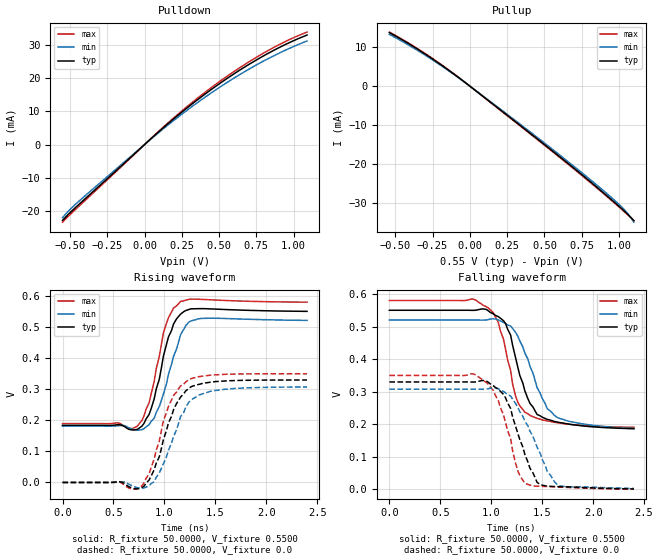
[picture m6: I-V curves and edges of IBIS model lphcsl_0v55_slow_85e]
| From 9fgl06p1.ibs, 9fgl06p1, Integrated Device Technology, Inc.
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[Model]   lphcsl_0v55_slow_85e
Model_type Output
Polarity   Inverting
Enable   Active-High
Vmeas =  0.4000V
Cref =   2.0000pF
Rref =   0.0
Vref =   0.4000V
C_comp   1.1000pF   1.0000pF   1.2000pF
[Temperature Range]   25.0000   85.0000   -40.0
[Voltage Range]   0.5500V   0.5200V   0.5800V
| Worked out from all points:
|   slope of the pulldown table from 0 to 0.083 V, typ, clamps not added: 24.5 ohm
|   slope of the pullup table from 0 to 0.083 V, typ, clamps not added: 33.4 ohm
|   rising waveform, R_fixture 50.0000, V_fixture 0.5500: 20-80 % time 164ps typ, 185ps min, 153ps max; typ from 0.184 V to 0.551 V
|   rising waveform, R_fixture 50.0000, V_fixture 0.0: 20-80 % time 212ps typ, 224ps min, 196ps max; typ from 0 V to 0.33 V
|   falling waveform, R_fixture 50.0000, V_fixture 0.5500: 20-80 % time 209ps typ, 258ps min, 182ps max; typ from 0.55 V to 0.186 V
|   falling waveform, R_fixture 50.0000, V_fixture 0.0: 20-80 % time 215ps typ, 272ps min, 192ps max; typ from 0.33 V to 0.002 V
[Pulldown]
|Voltage   I(typ)   I(min)   I(max)
-550mV    -22.86mA   -22.05mA   -23.4mA
-490mV    -20.12mA   -19.14mA   -20.7mA
-430mV    -17.63mA   -16.68mA   -18.17mA
50mV      2.058mA    1.922mA    2.135mA
230mV     9.045mA    8.465mA    9.373mA
410mV     15.37mA    14.42mA    15.91mA
590mV     21.04mA    19.77mA    21.74mA
770mV     26.03mA    24.5mA     26.86mA
930mV     29.87mA    28.16mA    30.76mA
1.09V     33.04mA    31.25mA    33.93mA
[Pullup]
|Voltage   I(typ)   I(min)   I(max)
-540mV    13.79mA    13.35mA    13.94mA
-360mV    9.757mA    9.424mA    9.891mA
-180mV    5.143mA    4.956mA    5.227mA
-20mV     596.4uA    573.5uA    607.4uA
340mV     -10.2mA    -9.898mA   -10.34mA
640mV     -19.35mA   -18.88mA   -19.54mA
920mV     -28.28mA   -27.72mA   -28.48mA
1.04V     -32.36mA   -32.02mA   -32.52mA
1.1V      -34.69mA   -35.06mA   -34.66mA
[Ramp]
| variable   typ   min   max
dV/dt_r  0.1981/0.2090n   0.1846/0.2327n   0.2101/0.1963n
dV/dt_f  0.2182/0.2310n   0.1998/0.2513n   0.2335/0.2061n
R_load = 50.0000
[Rising Waveform]
R_fixture= 50.0000
V_fixture= 0.5500
V_fixture_min= 0.5200
V_fixture_max= 0.5800
|time   V(typ)   V(min)   V(max)
0s        184mV      181.7mV    189.6mV
730ps     170.5mV    168.3mV    180.5mV
850ps     219.2mV    186.3mV    256.9mV
900ps     269.4mV    207.1mV    325.8mV
1.02ns    444.5mV    316.9mV    512.3mV
1.09ns    510.7mV    406.8mV    562.1mV
1.16ns    542.8mV    477.1mV    583.6mV
1.24ns    557.4mV    517mV      589.9mV
1.36ns    560.2mV    528.6mV    590.2mV
2.4ns     551.4mV    522.2mV    581mV
[Rising Waveform]
R_fixture= 50.0000
V_fixture= 0.0
V_fixture_min= 0.0
V_fixture_max= 0.0
|time   V(typ)   V(min)   V(max)
0s        0V         0V         0V
580ps     826.5uV    2.26mV     -2.284mV
700ps     -19.6mV    -13.42mV   -21.67mV
780ps     -16.64mV   -18.31mV   -10.91mV
900ps     41.24mV    2.869mV    75.98mV
1.04ns    192mV      104.4mV    244.9mV
1.12ns    254.6mV    169.8mV    291.5mV
1.24ns    302.9mV    258.8mV    331.7mV
1.55ns    326.1mV    298.5mV    347.8mV
2.4ns     330.1mV    307.6mV    350.1mV
[Falling Waveform]
R_fixture= 50.0000
V_fixture= 0.5500
V_fixture_min= 0.5200
V_fixture_max= 0.5800
|time   V(typ)   V(min)   V(max)
0s        550mV      520mV      580mV
820ps     549.7mV    520mV      584.4mV
1.07ns    530.3mV    520.6mV    512mV
1.19ns    473.7mV    501.6mV    365.3mV
1.24ns    402.5mV    481.5mV    285.3mV
1.33ns    302.2mV    418.6mV    237mV
1.45ns    230.1mV    312.6mV    218.2mV
1.55ns    215mV      247.5mV    210.2mV
1.65ns    206.8mV    220.7mV    204.8mV
2.4ns     186.4mV    187mV      190.8mV
[Falling Waveform]
R_fixture= 50.0000
V_fixture= 0.0
V_fixture_min= 0.0
V_fixture_max= 0.0
|time   V(typ)   V(min)   V(max)
0s        329.9mV    307.7mV    349.9mV
820ps     329.6mV    307.7mV    354.9mV
950ps     333.1mV    307.8mV    328.8mV
1.07ns    307.5mV    309.1mV    272mV
1.14ns    281.4mV    296.2mV    205.7mV
1.26ns    172.7mV    251.8mV    57.62mV
1.33ns    107.1mV    209.5mV    18.14mV
1.45ns    21.53mV    129.5mV    9.973mV
1.65ns    8.727mV    13.7mV     7.687mV
2.4ns     1.55mV     2.947mV    812.9uV
